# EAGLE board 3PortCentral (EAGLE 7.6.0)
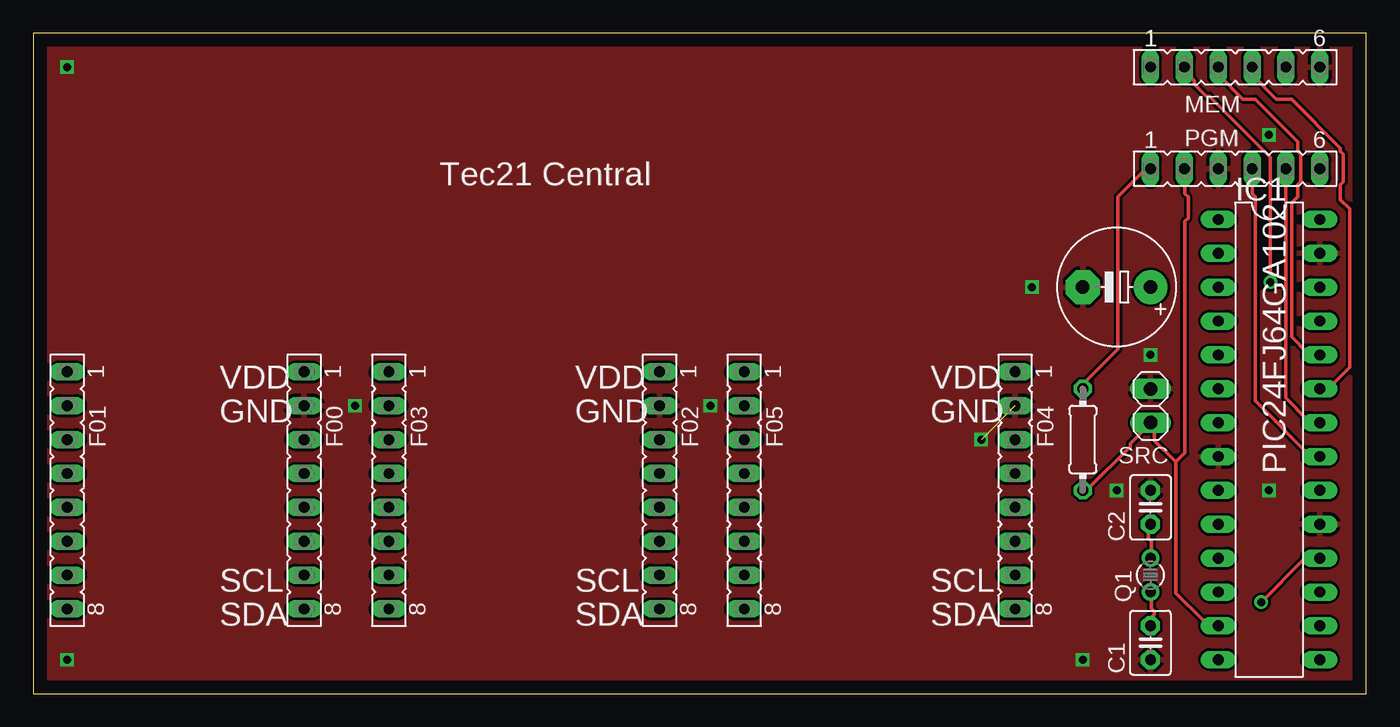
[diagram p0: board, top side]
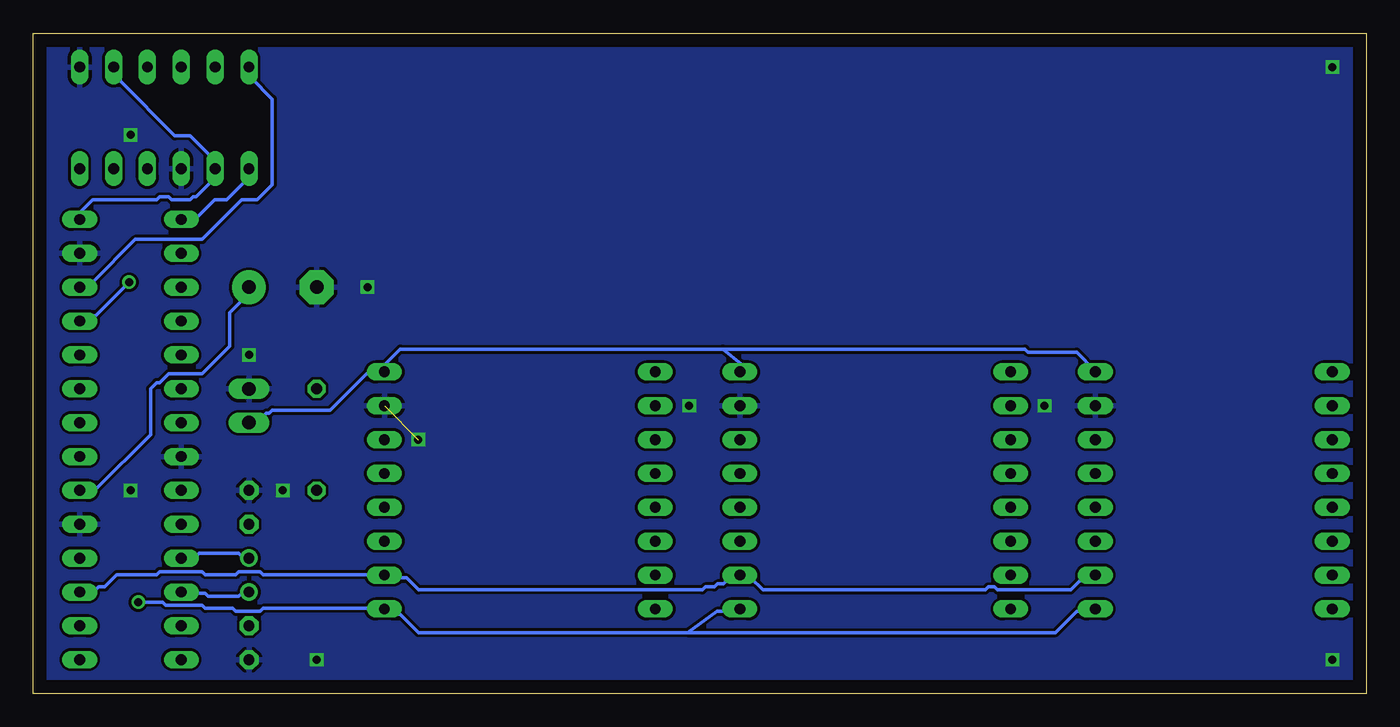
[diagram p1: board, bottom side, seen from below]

Size 100 x 49.52 mm. Coordinates in mm from the lower left corner, seen from the top.
Outline: 0,0 100,0 100,49.52 0,49.52 0,0
Copper layers (1*16): Top 0.035mm / dielectric 1.5mm / Bottom 0.035mm
Design rules "default": minimum track width 10mil, minimum drill 24mil, track to track 8mil, track to pad 8mil, pad to pad 8mil, via to via 8mil, smd to smd 8mil, copper to edge 40mil, drill to drill 8mil, minimum pad ring 10mil, minimum via ring 8mil, stop-mask expansion 4mil, vias tented up to drill 0mil, thermal gap 10mil

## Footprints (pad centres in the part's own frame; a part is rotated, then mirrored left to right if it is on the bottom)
C025-030X050 = drill 0.813 pad 1.422 octagon: 1 -1.27,0; 2 1.27,0
E5-8,5 = drill 1.016 pad 2.54: + -2.54,0 | drill 1.016 pad 2.54 octagon: - 2.54,0
FE08 = drill 0.813 long: 1 -8.89,0; 2 -6.35,0; 3 -3.81,0; 4 -1.27,0; 5 1.27,0; 6 3.81,0; 7 6.35,0; 8 8.89,0
DIL28-3 = drill 0.813 long: 1 -16.51,-3.81; 2 -13.97,-3.81; 3 -11.43,-3.81; 4 -8.89,-3.81; 5 -6.35,-3.81; 6 -3.81,-3.81; 7 -1.27,-3.81; 8 1.27,-3.81; 9 3.81,-3.81; 10 6.35,-3.81; 11 8.89,-3.81; 12 11.43,-3.81; 13 13.97,-3.81; 14 16.51,-3.81; 15 16.51,3.81; 16 13.97,3.81; 17 11.43,3.81; 18 8.89,3.81; 19 6.35,3.81; 20 3.81,3.81; 21 1.27,3.81; 22 -1.27,3.81; 23 -3.81,3.81; 24 -6.35,3.81; 25 -8.89,3.81; 26 -11.43,3.81; 27 -13.97,3.81; 28 -16.51,3.81
FE06 = drill 0.813 long: 1 -6.35,0; 2 -3.81,0; 3 -1.27,0; 4 1.27,0; 5 3.81,0; 6 6.35,0
TC26V = drill 0.813: 1 -1.27,0; 2 1.27,0
0204/7 = drill 0.813 octagon: 1 -3.81,0; 2 3.81,0
1X02 = drill 1.016 long: 1 -1.27,0; 2 1.27,0

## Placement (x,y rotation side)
C1  [C025-030X050]  83.82,3.81 90 top
C2  [C025-030X050]  83.82,13.97 270 top
C4  10uf  [E5-8,5]  81.28,30.48 180 top
F00  [FE08]  20.32,15.24 270 top
F01  [FE08]  2.54,15.24 270 top
F02  [FE08]  46.99,15.24 270 top
F03  [FE08]  26.67,15.24 270 top
F04  [FE08]  73.66,15.24 270 top
F05  [FE08]  53.34,15.24 270 top
IC1  PIC24FJ64GA002  [DIL28-3]  92.71,19.05 270 top
MEM  [FE06]  90.17,46.99 0 top
PGM  [FE06]  90.17,39.37 0 top
Q1  [TC26V]  83.82,8.89 90 top
R1  10k  [0204/7]  78.74,19.05 270 top
SRC  [1X02]  83.82,21.59 90 top

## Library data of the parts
C1 C2 C4 = adafruit
F00 F01-F05 MEM PGM = con-lsta; OC_FARNELL: unknown; OC_NEWARK: unknown
IC1 = microchip; MPN: PIC24FJ64GA002-I/SP; OC_FARNELL: 1332298; OC_NEWARK: 88K6132
Q1 = crystal; OC_FARNELL: unknown; OC_NEWARK: unknown
R1 = resistor
SRC = pinhead

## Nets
GND: C1.1 C2.1 C4.- F00.2 F02.2 F04.2 IC1.8 IC1.19 IC1.27 MEM.6 PGM.3 SRC.2
MISO: IC1.23 MEM.4
MOSI: IC1.24 MEM.3
N$1: IC1.1 PGM.1 R1.1
N$2: C1.2 IC1.12 Q1.1
N$3: C2.2 IC1.11 Q1.2
N$4: IC1.21 PGM.4
N$5: IC1.22 PGM.5
N$6: C4.+ IC1.20
SCL: F00.7 F02.7 F04.7 IC1.17
SDA: F00.8 F02.8 F04.8 IC1.18
SPICK: IC1.25 MEM.2
SS: IC1.26 MEM.1
VDD: F00.1 F02.1 F04.1 IC1.13 IC1.28 MEM.5 PGM.2 R1.2 SRC.1

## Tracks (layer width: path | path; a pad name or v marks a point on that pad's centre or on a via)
GND  (via drill 0.6)  (1 unrouted)
  other vias: 2.54,2.54 2.54,46.99 74.93,30.48 83.82,25.4 78.74,2.54 81.28,15.24 92.71,15.24 92.71,41.91 24.13,21.59 50.8,21.59 71.12,19.05
  pour Top: -1.27,50.8 101.6,50.8 101.6,-1.27 -1.27,-1.27
  pour Bottom: -1.27,50.8 101.6,50.8 101.6,-1.27 -1.27,-1.27
MISO
  Top 0.254: MEM.4 91.44,46.41 93.27,44.58 94.41,44.58 98.07,40.92 98.07,40.69 98.3,40.46 98.3,38.41 98.07,38.18 98.07,37.03 98.75,36.35 98.75,24.46 97.61,23.32 97.16,23.32 96.7,22.86 IC1.23
MOSI
  Top 0.254: IC1.24 96.47,25.6 95.56,25.6 94.41,26.75 94.41,36.8 94.87,37.26 94.87,38.18 95.1,38.41 95.1,40.46 94.87,40.69 94.87,41.38 91.67,44.58 90.75,44.58 88.92,46.41 88.92,46.86 MEM.3
N$1
  Top 0.254: R1.1 78.87,22.86 78.87,23.32 81.38,25.83 81.38,37.26 83.67,39.55 PGM.1
  Bottom 0.254: IC1.1 88.7,35.66 87.78,35.66 86.41,37.03 85.5,37.03 83.9,38.63 83.9,39.32 PGM.1
N$2
  Top 0.254: Q1.1 83.9,7.54 83.9,6.4 84.12,6.17 84.12,5.94 83.9,5.71 83.9,5.26 C1.2
  Bottom 0.254: IC1.12 88.7,7.54 87.1,7.54 86.87,7.32 84.58,7.32 84.35,7.54 83.9,7.54 Q1.1
N$3
  Top 0.254: Q1.2 83.9,10.29 83.9,11.43 83.67,11.66 83.67,12.57 C2.2
  Bottom 0.254: IC1.11 88.7,10.29 87.78,10.29 87.55,10.52 84.58,10.52 84.35,10.29 83.9,10.29 Q1.2
N$4
  Top 0.254: PGM.4 91.44,37.49 91.67,37.26 91.67,21.95 95.56,18.06 95.56,17.83 96.47,17.83 IC1.21
N$5
  Top 0.254: IC1.22 96.47,20.34 95.56,20.34 95.56,20.57 93.95,22.17 93.95,39.32 PGM.5
N$6
  Bottom 0.254: IC1.20 96.47,15.32 95.33,15.32 91.21,19.43 91.21,22.86 90.75,23.32 90.53,23.32 89.84,24 87.33,24 85.27,26.06 85.27,28.57 83.9,29.95 83.9,30.4 C4.+
SCL
  Bottom 0.254: IC1.17 96.47,7.77 95.33,7.77 95.1,8 94.64,8 93.73,8.91 90.75,8.91 90.53,9.14 87.33,9.14 87.1,8.91 84.81,8.91 84.58,9.14 82.98,9.14 82.75,8.91 73.84,8.91 F04.7 73.61,8.69 72.01,8.69 71.09,7.77 49.81,7.77 49.58,8 48.9,8 48.67,8.23 48.23,8.23 47.78,8.69 47.09,8.69 F02.7 46.86,8.69 46.18,8.69 45.26,7.77 28.57,7.77 28.35,8 27.89,8 27.66,7.77 22.17,7.77 21.49,8.46 20.57,8.46 20.34,8.69 F00.7
SDA  (via drill 0.61)
  Top 0.254: v92.13,6.86 95.33,10.06 96.47,10.06 IC1.18
  Bottom 0.254: 50.93,4.57 23.32,4.57 21.72,6.17 20.34,6.17 F00.8 | 50.93,4.57 48.72,6.17 48.13,6.17 F02.8 | 50.93,4.57 71.09,4.57 72.47,5.94 73.38,5.94 73.61,6.17 F04.8 73.84,6.4 82.75,6.4 82.98,6.17 84.81,6.17 85.04,6.4 87.1,6.4 87.33,6.63 90.07,6.63 90.3,6.86 v92.13,6.86
SPICK  (via drill 0.61)
  Top 0.254: v92.81,30.86 92.81,40.23 88.24,44.81 88.01,44.81 87.1,45.72 87.1,45.95 86.41,46.63 86.41,46.86 MEM.2
  Bottom 0.254: v92.81,30.86 95.33,28.35 96.24,28.35 96.47,28.12 IC1.25
SS
  Bottom 0.254: IC1.26 96.47,30.63 96.24,30.86 95.56,30.86 92.35,34.06 87.33,34.06 84.35,37.03 83.21,37.03 82.07,38.18 82.07,44.58 83.67,46.18 83.67,46.86 MEM.1
VDD
  Top 0.254: R1.2 78.87,15.32 79.1,15.32 82.3,18.52 82.3,18.75 83.67,20.12 SRC.1 83.9,20.12 84.12,19.89 84.12,18.97 85.72,17.37 | 85.72,17.37 85.72,7.54 87.78,5.49 87.78,5.26 88.7,5.26 IC1.13 | 85.72,17.37 86.41,18.06 86.41,35.43 86.64,35.66 86.64,37.26 86.41,37.49 86.41,39.32 PGM.2
  Bottom 0.254: 48.26,25.83 25.6,25.83 25.38,25.6 21.72,25.6 20.34,24.23 F00.1 | 48.26,25.83 46.86,24.69 46.86,24.23 F02.1 | IC1.28 96.47,35.66 96.47,36.12 95.56,37.03 90.75,37.03 90.53,37.26 89.84,37.26 89.61,37.03 88.24,37.03 88.01,37.26 87.78,37.26 86.64,38.41 86.41,38.41 86.41,39.32 PGM.2 86.41,39.55 86.41,40.01 88.24,41.83 89.38,41.83 93.5,45.95 93.5,46.41 93.95,46.86 MEM.5 | SRC.1 83.67,20.34 83.21,20.34 82.53,21.03 82.3,21.03 82.07,21.26 77.72,21.26 74.98,24 73.84,24 F04.1 73.61,24.23 73.61,24.69 72.47,25.83 48.26,25.83

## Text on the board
tPlace: Tec21 Central | VDD | VDD | VDD | GND | GND | GND | PIC24FJ64GA102 | SCL | SCL | SCL | SDA | SDA | SDA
